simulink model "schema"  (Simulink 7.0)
settings: Solver=ode23  StartTime=0.0  StopTime=200  RelTol=1e-3

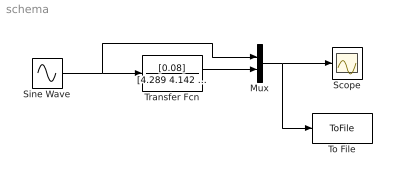
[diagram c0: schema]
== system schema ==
  Mux : Mux  Inputs=2
  Scope : Scope
  Sine Wave : Sin  Frequency=0.05  SampleTime=0
  To File : ToFile  Filename=Sinusovky.mat
  Transfer Fcn : TransferFcn  Numerator=[0.08]  Denominator=[4.289 4.142 1]
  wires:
  Sine Wave/1 -> Mux/1, Transfer Fcn/1
  Mux/1 -> Scope/1, To File/1
  Transfer Fcn/1 -> Mux/2
